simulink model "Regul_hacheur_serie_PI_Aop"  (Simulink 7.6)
settings: Solver=ode23tb  StartTime=0.0  StopTime=100  RelTol=1e-3
InitFcn:
  | clc, close all, clear all
  | rc=30;
  | 
  | Kp=1e-5; %1e-5 marche
  | R1=10e3;
  | R2=Kp*R1;
  | Ti=1e-4;
  | C=Ti/R2;
StopFcn:
  | clc
  | close all, clc
  | 
  | load csg_Imoy_charge.mat
  | figure
  | plot(x(1,:),x(2,:),x(1,:),x(3,:),x(1,:),x(4,:))
  | xlabel('temps')
  | title('Courant charge et Consigne')
  | grid
  | 
  | load err-cde-PID.mat
  | figure
  | plotyy(y(1,:),y(2,:),y(1,:),y(3,:))
  | xlabel('temps')
  | title('Erreur et Commande')
  | grid
  | 
  | delete *.mat
libraries: fl_lib x27, nesl_utility x13, powerlib x10, elec_lib x10, powerlib_extras x1

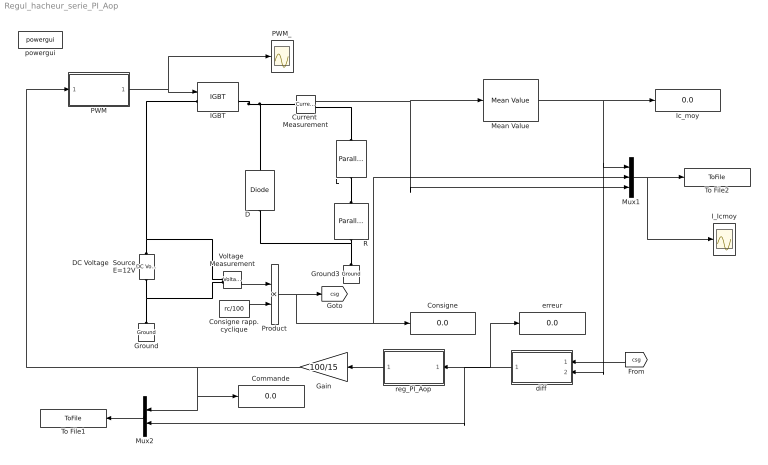
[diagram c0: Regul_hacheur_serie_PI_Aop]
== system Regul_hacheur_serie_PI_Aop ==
  Commande : Display
  Consigne : Display
  Consigne rapp. cyclique : Constant  Value=rc/100
  Current  Measurement : powerlib/Measurements/Current Measurement  DialogController=POWERSYS.PowerSysDialog  SystemSampleTime=-1  PhasorSimulation=off  OutputType=Complex  PSBequivalent=0
  D : powerlib/Power Electronics/Diode  DialogController=POWERSYS.PowerSysDialog  SystemSampleTime=-1  Ron=0.001  Lon=0  Vf=0.7  IC=0  UseSnubber=off  Rs=1e12  Cs=250e-12  Measurements=off
  DC Voltage  Source E=12V : powerlib/Electrical Sources/DC Voltage Source  DialogController=POWERSYS.PowerSysDialog  SystemSampleTime=-1  Amplitude=12  Measurements=None
  Gain : Gain  Gain=100/15
  Ground : powerlib/Elements/Ground  DialogController=POWERSYS.PowerSysDialog  PhysicalDomain=powersysdomain  SubClassName=unknown  LeftPortType=p1  RightPortType=p1  LConnTagsString=a
  Ground3 : powerlib/Elements/Ground  DialogController=POWERSYS.PowerSysDialog  PhysicalDomain=powersysdomain  SubClassName=unknown  LeftPortType=p1  RightPortType=p1  LConnTagsString=a
  IGBT : powerlib/Power Electronics/IGBT  DialogController=POWERSYS.PowerSysDialog  SystemSampleTime=-1  Ron=0.001  Lon=0  Vf=1  Tf=1e-6  Tt=2e-6  IC=0  Rs=1e5  Cs=inf  Measurements=on
  I_Icmoy : Scope
  Ic_moy : Display
  L : powerlib/Elements/Parallel RLC Branch  DialogController=POWERSYS.PowerSysDialog  PhysicalDomain=powersysdomain  SubClassName=unknown  LeftPortType=p1  RightPortType=p1  LConnTagsString=a  RConnTagsString=__new0  BranchType=L  Resistance=50  Inductance=10  SetiL0=off  InitialCurrent=0  Capacitance=25e-06  Setx0=off  InitialVoltage=0  Measurements=Branch voltage and current
  Mean Value : powerlib_extras/Measurements/Mean Value  DialogController=POWERSYS.PowerSysDialog  SystemSampleTime=-1  Period=10
  Mux1 : Mux  Inputs=3
  Mux2 : Mux  Inputs=2
  PWM : Subsystem
  PWM_ : Scope
  Product : Product
  R : powerlib/Elements/Parallel RLC Branch  DialogController=POWERSYS.PowerSysDialog  PhysicalDomain=powersysdomain  SubClassName=unknown  LeftPortType=p1  RightPortType=p1  LConnTagsString=a  RConnTagsString=__new0  BranchType=R  Resistance=1  Inductance=1.0  SetiL0=off  InitialCurrent=0  Capacitance=25e-06  Setx0=off  InitialVoltage=0  Measurements=Branch voltage and current
  To File1 : ToFile  Filename=err-cde-PID  MatrixName=y
  To File2 : ToFile  Filename=csg_Imoy_charge  MatrixName=x
  Voltage  Measurement : powerlib/Measurements/Voltage Measurement  DialogController=POWERSYS.PowerSysDialog  SystemSampleTime=-1  PhasorSimulation=off  OutputType=Complex  PSBequivalent=0
  diff : Subsystem
  erreur : Display
  powergui : powerlib/powergui  SystemSampleTime=-1  SimulationMode=Continuous  SampleTime=0  frequency=60  SPID=off  DisableSnubberDevices=off  DisableRonSwitches=off  DisableVfSwitches=off  SwTol=0  Interpol=off  frequencyindice=0  echomessages=off  HookPort=off  DisplayEquations=off  FunctionMessages=off  EnableUseOfTLC=off  x0status=blocks  RestoreLinks=warning  ResistiveCurrentMeasurement=off  Frange=[0:2:500]  Ylog=off  Xlog=on  ShowGrid=off  save=off  variable=ZData  ZoomFFT=on  StartTime=0.0  cycles=1  DisplayStyle=1  fundamental=60  FreqAxis=off  MaxFrequency=1000  frequencyindicesteady=1  RmsSteady=1  display=off  Ts=0  methode=off
  reg_PI_Aop : Subsystem
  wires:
  PWM/1(PWM) -> PWM_/1, IGBT/1
  Current  Measurement/1 -> Mean Value/1, Mux1/3
  Mean Value/1 -> Ic_moy/1, Mux1/1, diff/2(-I)
  Mux1/1 -> To File2/1, I_Icmoy/1
  Voltage  Measurement/1 -> Product/1
  Product/1 -> [csg], Consigne/1, Mux1/2
  Consigne rapp. cyclique/1 -> Product/2
  diff/1(err) -> erreur/1, Mux2/2, reg_PI_Aop/1(err)
  reg_PI_Aop/1(cde) -> Gain/1
  Mux2/1 -> To File1/1
  [csg] -> diff/1(+Csg)
  Gain/1 -> PWM/1(rc (%)), Commande/1, Mux2/1
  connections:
  DC Voltage  Source E=12V/LConn1 -- Ground/LConn1 -- Voltage  Measurement/LConn2
  DC Voltage  Source E=12V/RConn1 -- IGBT/LConn1 -- Voltage  Measurement/LConn1
  R/RConn1 -- Ground3/LConn1 -- D/LConn1
  IGBT/RConn1 -- D/RConn1 -- Current  Measurement/LConn1
  L/RConn1 -- R/LConn1
  L/LConn1 -- Current  Measurement/RConn1

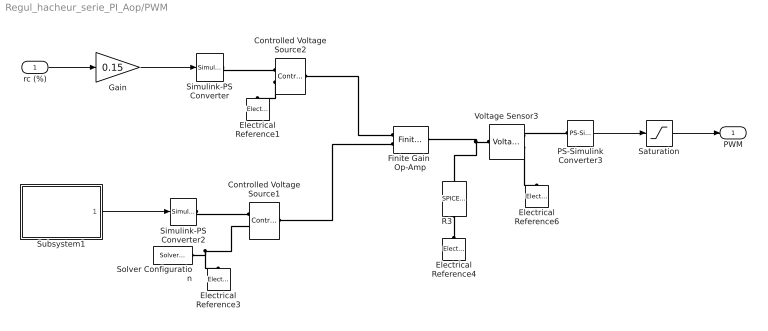
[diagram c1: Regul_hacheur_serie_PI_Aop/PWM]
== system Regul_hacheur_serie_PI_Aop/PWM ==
  rc (%) : Inport
  Controlled Voltage Source1 : fl_lib/Electrical/Electrical Sources/Controlled Voltage Source  DialogController=NetworkEngine.DynNeDlgSource  SystemSampleTime=-1  i_Log=off  v_Log=off  LocalVarNames=|current|voltage|power  LocalVarDescs=|Current (A)|Voltage (V)|Power (W)  LocalVarLogging=[0 0 0]
  Controlled Voltage Source2 : fl_lib/Electrical/Electrical Sources/Controlled Voltage Source  DialogController=NetworkEngine.DynNeDlgSource  SystemSampleTime=-1  i_Log=off  v_Log=off  LocalVarNames=|current|voltage|power  LocalVarDescs=|Current (A)|Voltage (V)|Power (W)  LocalVarLogging=[0 0 0]
  Electrical Reference{1,3..4,6} (4 alike) : fl_lib/Electrical/Electrical Elements/Electrical Reference  DialogController=NetworkEngine.DynNeDlgSource  SystemSampleTime=-1  i_Log=off  LocalVarNames=|i  LocalVarDescs=|i  LocalVarLogging=[]
  Finite Gain  Op-Amp : elec_lib/Integrated Circuits/Finite Gain Op-Amp  DialogController=NetworkEngine.DynNeDlgSource  SystemSampleTime=-1  A=1000  Rin=1e+06 Ohm  Rout=100 Ohm  Vmin=-12 V  Vmax=12 V  LocalVarNames=|power  LocalVarDescs=|Dissipated power (W)  LocalVarLogging=0
  Gain : Gain  Gain=0.15
  PS-Simulink Converter3 : nesl_utility/PS-Simulink Converter  DialogController=NetworkEngine.DynNeUtilDlgSource  SystemSampleTime=-1  PhysicalDomain=network_engine_domain  LeftPortType=input  RightPortType=output  SubClassName=ps_output  Unit=1  AffineConversion=off
  R3 : elec_lib/Additional Components/SPICE-Compatible Components/Passive Devices/SPICE Resistor  DialogController=NetworkEngine.DynNeDlgSource  SystemSampleTime=-1  SCALE=1  R_param=1  R=10e3 Ohm  RSH=0 Ohm  LENGTH=1e-06 m  WIDTH=1e-06 m  NARROW=0 m  T_param=1  TC1=0 1/K  TC2=0 1/K^2  TOFFSET=0 K  TFIXED=300.15 K  TMEAS=300.15 K  LocalVarLogging=[]
  Saturation : Saturate  UpperLimit=1  LowerLimit=0
  Simulink-PS Converter : nesl_utility/Simulink-PS Converter  DialogController=NetworkEngine.DynNeUtilDlgSource  SystemSampleTime=-1  PhysicalDomain=network_engine_domain  LeftPortType=input  RightPortType=output  SubClassName=ps_input  Unit=1  AffineConversion=off  InputFilterTimeConstant=.001  UdotUserProvided=0
  Simulink-PS Converter2 : nesl_utility/Simulink-PS Converter  DialogController=NetworkEngine.DynNeUtilDlgSource  SystemSampleTime=-1  PhysicalDomain=network_engine_domain  LeftPortType=input  RightPortType=output  SubClassName=ps_input  Unit=1  AffineConversion=off  InputFilterTimeConstant=.001  UdotUserProvided=0
  Solver Configuration : nesl_utility/Solver Configuration  DialogController=NetworkEngine.DynNeUtilDlgSource  SystemSampleTime=-1  PhysicalDomain=network_engine_domain  LeftPortType=input  RightPortType=generic  SubClassName=solver  Accelerate=off  Profile=off  ResidualTolerance=1e-12  MaxNonlinIter=12  MaxModeIter=2  DoFixedCost=on  UseLocalSampling=off  DoDC=off  LinearAlgebra=Sparse  LocalSolverSampleTime=.001  LocalSolverChoice=NE_BACKWARD_EULER_ADVANCER  UseLocalSolver=off
  Subsystem1 : Subsystem
  Voltage Sensor3 : fl_lib/Electrical/Electrical Sensors/Voltage Sensor  DialogController=NetworkEngine.DynNeDlgSource  SystemSampleTime=-1  i1_Log=off  v1_Log=off  LocalVarNames=|i1|v1  LocalVarDescs=|i1|v1  LocalVarLogging=[]
  PWM : Outport
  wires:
  Gain/1 -> Simulink-PS Converter/1
  Saturation/1 -> PWM/1
  PS-Simulink Converter3/1 -> Saturation/1
  rc (%)/1 -> Gain/1
  Subsystem1/1(tri) -> Simulink-PS Converter2/1
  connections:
  Voltage Sensor3/RConn1 -- PS-Simulink Converter3/LConn1
  Voltage Sensor3/LConn1 -- R3/RConn1 -- Finite Gain  Op-Amp/RConn1
  Voltage Sensor3/RConn2 -- Electrical Reference6/LConn1
  Electrical Reference4/LConn1 -- R3/LConn1
  Controlled Voltage Source2/RConn2 -- Electrical Reference1/LConn1
  Simulink-PS Converter/RConn1 -- Controlled Voltage Source2/RConn1
  Finite Gain  Op-Amp/LConn1 -- Controlled Voltage Source2/LConn1
  Solver Configuration/RConn1 -- Electrical Reference3/LConn1 -- Controlled Voltage Source1/RConn2
  Simulink-PS Converter2/RConn1 -- Controlled Voltage Source1/RConn1
  Controlled Voltage Source1/LConn1 -- Finite Gain  Op-Amp/LConn2

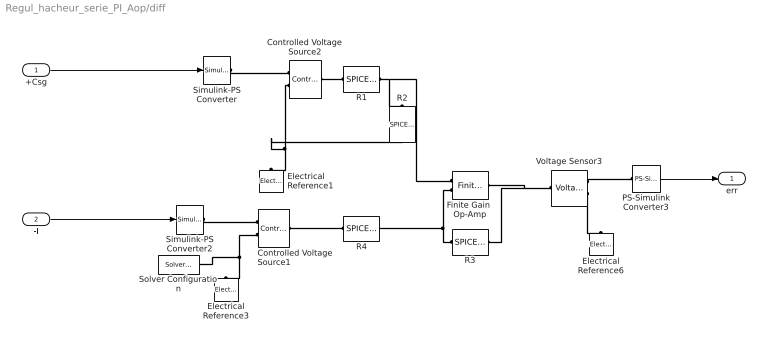
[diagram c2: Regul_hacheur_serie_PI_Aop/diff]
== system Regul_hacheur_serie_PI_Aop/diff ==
  +Csg : Inport
  -I : Inport  Port=2
  Controlled Voltage Source1 : fl_lib/Electrical/Electrical Sources/Controlled Voltage Source  DialogController=NetworkEngine.DynNeDlgSource  SystemSampleTime=-1  i_Log=off  v_Log=off  LocalVarNames=|current|voltage|power  LocalVarDescs=|Current (A)|Voltage (V)|Power (W)  LocalVarLogging=[0 0 0]
  Controlled Voltage Source2 : fl_lib/Electrical/Electrical Sources/Controlled Voltage Source  DialogController=NetworkEngine.DynNeDlgSource  SystemSampleTime=-1  i_Log=off  v_Log=off  LocalVarNames=|current|voltage|power  LocalVarDescs=|Current (A)|Voltage (V)|Power (W)  LocalVarLogging=[0 0 0]
  Electrical Reference1 : fl_lib/Electrical/Electrical Elements/Electrical Reference  DialogController=NetworkEngine.DynNeDlgSource  SystemSampleTime=-1  i_Log=off  LocalVarNames=|i  LocalVarDescs=|i  LocalVarLogging=[]
  Electrical Reference3 : fl_lib/Electrical/Electrical Elements/Electrical Reference  DialogController=NetworkEngine.DynNeDlgSource  SystemSampleTime=-1  i_Log=off  LocalVarNames=|i  LocalVarDescs=|i  LocalVarLogging=[]
  Electrical Reference6 : fl_lib/Electrical/Electrical Elements/Electrical Reference  DialogController=NetworkEngine.DynNeDlgSource  SystemSampleTime=-1  i_Log=off  LocalVarNames=|i  LocalVarDescs=|i  LocalVarLogging=[]
  Finite Gain  Op-Amp : elec_lib/Integrated Circuits/Finite Gain Op-Amp  DialogController=NetworkEngine.DynNeDlgSource  SystemSampleTime=-1  A=1000  Rin=1e+06 Ohm  Rout=100 Ohm  Vmin=-12 V  Vmax=12 V  LocalVarNames=|power  LocalVarDescs=|Dissipated power (W)  LocalVarLogging=0
  PS-Simulink Converter3 : nesl_utility/PS-Simulink Converter  DialogController=NetworkEngine.DynNeUtilDlgSource  SystemSampleTime=-1  PhysicalDomain=network_engine_domain  LeftPortType=input  RightPortType=output  SubClassName=ps_output  Unit=1  AffineConversion=off
  R{1..4} (4 alike) : elec_lib/Additional Components/SPICE-Compatible Components/Passive Devices/SPICE Resistor  DialogController=NetworkEngine.DynNeDlgSource  SystemSampleTime=-1  SCALE=1  R_param=1  R=10e3 Ohm  RSH=0 Ohm  LENGTH=1e-06 m  WIDTH=1e-06 m  NARROW=0 m  T_param=1  TC1=0 1/K  TC2=0 1/K^2  TOFFSET=0 K  TFIXED=300.15 K  TMEAS=300.15 K  LocalVarLogging=[]
  Simulink-PS Converter : nesl_utility/Simulink-PS Converter  DialogController=NetworkEngine.DynNeUtilDlgSource  SystemSampleTime=-1  PhysicalDomain=network_engine_domain  LeftPortType=input  RightPortType=output  SubClassName=ps_input  Unit=1  AffineConversion=off  InputFilterTimeConstant=.001  UdotUserProvided=0
  Simulink-PS Converter2 : nesl_utility/Simulink-PS Converter  DialogController=NetworkEngine.DynNeUtilDlgSource  SystemSampleTime=-1  PhysicalDomain=network_engine_domain  LeftPortType=input  RightPortType=output  SubClassName=ps_input  Unit=1  AffineConversion=off  InputFilterTimeConstant=.001  UdotUserProvided=0
  Solver Configuration : nesl_utility/Solver Configuration  DialogController=NetworkEngine.DynNeUtilDlgSource  SystemSampleTime=-1  PhysicalDomain=network_engine_domain  LeftPortType=input  RightPortType=generic  SubClassName=solver  Accelerate=off  Profile=off  ResidualTolerance=1e-12  MaxNonlinIter=12  MaxModeIter=2  DoFixedCost=on  UseLocalSampling=off  DoDC=off  LinearAlgebra=Sparse  LocalSolverSampleTime=.001  LocalSolverChoice=NE_BACKWARD_EULER_ADVANCER  UseLocalSolver=off
  Voltage Sensor3 : fl_lib/Electrical/Electrical Sensors/Voltage Sensor  DialogController=NetworkEngine.DynNeDlgSource  SystemSampleTime=-1  i1_Log=off  v1_Log=off  LocalVarNames=|i1|v1  LocalVarDescs=|i1|v1  LocalVarLogging=[]
  err : Outport
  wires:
  -I/1 -> Simulink-PS Converter2/1
  +Csg/1 -> Simulink-PS Converter/1
  PS-Simulink Converter3/1 -> err/1
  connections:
  Simulink-PS Converter2/RConn1 -- Controlled Voltage Source1/RConn1
  Controlled Voltage Source1/RConn2 -- Electrical Reference3/LConn1 -- Solver Configuration/RConn1
  Simulink-PS Converter/RConn1 -- Controlled Voltage Source2/RConn1
  Controlled Voltage Source2/RConn2 -- Electrical Reference1/LConn1 -- R2/RConn1
  Voltage Sensor3/RConn2 -- Electrical Reference6/LConn1
  R3/RConn1 -- Finite Gain  Op-Amp/RConn1 -- Voltage Sensor3/LConn1
  Voltage Sensor3/RConn1 -- PS-Simulink Converter3/LConn1
  R1/LConn1 -- Controlled Voltage Source2/LConn1
  R1/RConn1 -- R2/LConn1 -- Finite Gain  Op-Amp/LConn1
  R3/LConn1 -- Finite Gain  Op-Amp/LConn2 -- R4/RConn1
  Controlled Voltage Source1/LConn1 -- R4/LConn1

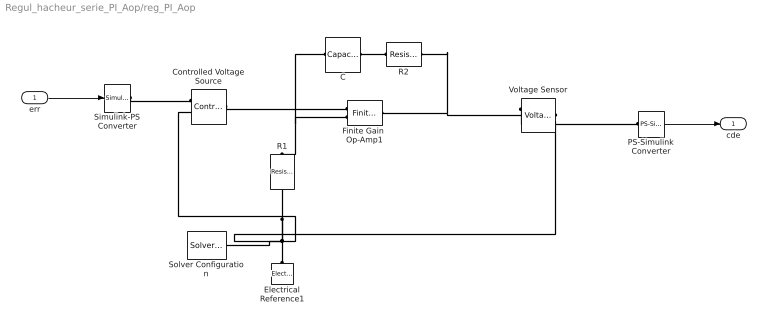
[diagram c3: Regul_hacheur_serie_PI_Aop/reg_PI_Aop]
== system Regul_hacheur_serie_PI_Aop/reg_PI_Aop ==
  err : Inport
  C : fl_lib/Electrical/Electrical Elements/Capacitor  DialogController=NetworkEngine.DynNeDlgSource  SystemSampleTime=-1  c=C F  v0=0 V  r=1e-6 Ohm  g=0 1/Ohm  i_Log=off  v_Log=off  vc_Log=off  LocalVarNames=|i|v|vc  LocalVarDescs=|i|v|Internal variable for voltage across capacitor term  LocalVarLogging=[0 0 0]
  Controlled Voltage Source : fl_lib/Electrical/Electrical Sources/Controlled Voltage Source  DialogController=NetworkEngine.DynNeDlgSource  SystemSampleTime=-1  i_Log=off  v_Log=off  LocalVarNames=|i|v  LocalVarDescs=|i|v  LocalVarLogging=[0 0]
  Electrical Reference1 : fl_lib/Electrical/Electrical Elements/Electrical Reference  DialogController=NetworkEngine.DynNeDlgSource  SystemSampleTime=-1  i_Log=off  LocalVarNames=|i  LocalVarDescs=|i  LocalVarLogging=[]
  Finite Gain  Op-Amp1 : elec_lib/Integrated Circuits/Finite Gain Op-Amp  DialogController=NetworkEngine.DynNeDlgSource  SystemSampleTime=-1  A=1000  Rin=1e+6 Ohm  Rout=100 Ohm  Vmin=-15 V  Vmax=15 V  LocalVarLogging=[]
  PS-Simulink Converter : nesl_utility/PS-Simulink Converter  DialogController=NetworkEngine.DynNeUtilDlgSource  SystemSampleTime=-1  PhysicalDomain=network_engine_domain  LeftPortType=input  RightPortType=output  SubClassName=ps_output  Unit=1  AffineConversion=off
  R1 : fl_lib/Electrical/Electrical Elements/Resistor  DialogController=NetworkEngine.DynNeDlgSource  SystemSampleTime=-1  R=R1 Ohm  i_Log=off  v_Log=off  LocalVarNames=|current|voltage|power  LocalVarDescs=|Resistor current (A)|Voltage across resistor (V)|Power (W)  LocalVarLogging=[0 0 0]
  R2 : fl_lib/Electrical/Electrical Elements/Resistor  DialogController=NetworkEngine.DynNeDlgSource  SystemSampleTime=-1  R=R2 Ohm  i_Log=off  v_Log=off  LocalVarNames=|current|voltage|power  LocalVarDescs=|Resistor current (A)|Voltage across resistor (V)|Power (W)  LocalVarLogging=[0 0 0]
  Simulink-PS Converter : nesl_utility/Simulink-PS Converter  DialogController=NetworkEngine.DynNeUtilDlgSource  SystemSampleTime=-1  PhysicalDomain=network_engine_domain  LeftPortType=input  RightPortType=output  SubClassName=ps_input  Unit=1  AffineConversion=off  InputFilterTimeConstant=.001  UdotUserProvided=0
  Solver Configuration : nesl_utility/Solver Configuration  DialogController=NetworkEngine.DynNeUtilDlgSource  SystemSampleTime=-1  PhysicalDomain=network_engine_domain  LeftPortType=input  RightPortType=generic  SubClassName=solver  Accelerate=off  Profile=off  ResidualTolerance=1e-9  MaxNonlinIter=3  MaxModeIter=2  DoFixedCost=off  UseLocalSampling=off  DoDC=off  LinearAlgebra=Sparse  LocalSolverSampleTime=.001  LocalSolverChoice=NE_BACKWARD_EULER_ADVANCER  UseLocalSolver=off
  Voltage Sensor : fl_lib/Electrical/Electrical Sensors/Voltage Sensor  DialogController=NetworkEngine.DynNeDlgSource  SystemSampleTime=-1  i1_Log=off  v1_Log=off  LocalVarNames=|i1|v1  LocalVarDescs=|i1|v1  LocalVarLogging=[0 0]
  cde : Outport
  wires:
  PS-Simulink Converter/1 -> cde/1
  err/1 -> Simulink-PS Converter/1
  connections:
  C/LConn1 -- R1/RConn1 -- Finite Gain  Op-Amp1/LConn2
  C/RConn1 -- R2/LConn1
  R1/LConn1 -- Voltage Sensor/RConn2 -- Controlled Voltage Source/RConn2 -- Electrical Reference1/LConn1 -- Solver Configuration/RConn1
  Finite Gain  Op-Amp1/RConn1 -- R2/RConn1 -- Voltage Sensor/LConn1
  Voltage Sensor/RConn1 -- PS-Simulink Converter/LConn1
  Simulink-PS Converter/RConn1 -- Controlled Voltage Source/RConn1
  Controlled Voltage Source/LConn1 -- Finite Gain  Op-Amp1/LConn1

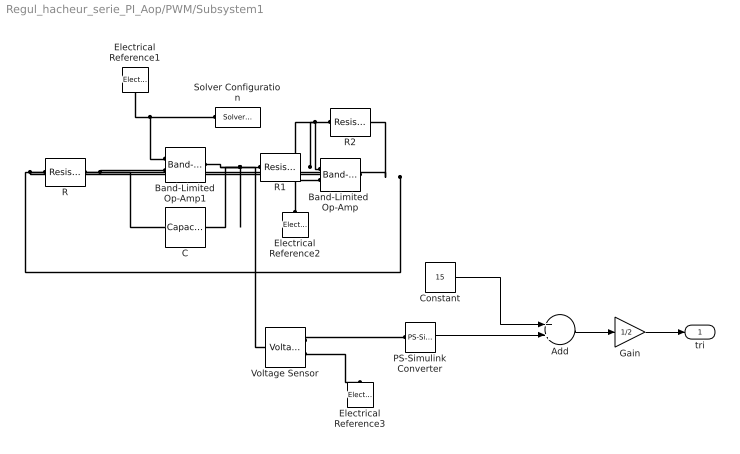
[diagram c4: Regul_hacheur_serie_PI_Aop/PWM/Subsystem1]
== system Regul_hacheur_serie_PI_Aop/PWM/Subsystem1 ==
  Add : Sum
  Band-Limited  Op-Amp : elec_lib/Integrated Circuits/Band-Limited Op-Amp  DialogController=NetworkEngine.DynNeDlgSource  SystemSampleTime=-1  A=1000  Rin=1e+06 Ohm  Rout=100 Ohm  Vmin=-15 V  Vmax=15 V  Vdotmax=1000 V/s  f=1e+05 Hz  V0=0 V  LocalVarNames=|power  LocalVarDescs=|Dissipated power (W)  LocalVarLogging=0
  Band-Limited Op-Amp1 : elec_lib/Integrated Circuits/Band-Limited Op-Amp  DialogController=NetworkEngine.DynNeDlgSource  SystemSampleTime=-1  A=1000  Rin=1e+06 Ohm  Rout=100 Ohm  Vmin=-15 V  Vmax=15 V  Vdotmax=1000 V/s  f=1e+05 Hz  V0=0 V  LocalVarNames=|power  LocalVarDescs=|Dissipated power (W)  LocalVarLogging=0
  C : fl_lib/Electrical/Electrical Elements/Capacitor  DialogController=NetworkEngine.DynNeDlgSource  SystemSampleTime=-1  c=0.1e-5 F  v0=0.1 V  r=1e-6 Ohm  g=0 1/Ohm  i_Log=off  v_Log=off  vc_Log=off  LocalVarNames=|current|voltage|power  LocalVarDescs=|Capacitor current (A)|Voltage across capacitor (V)|Power (W)  LocalVarLogging=[0 0 0]
  Constant : Constant  Value=15
  Electrical Reference1 : fl_lib/Electrical/Electrical Elements/Electrical Reference  DialogController=NetworkEngine.DynNeDlgSource  SystemSampleTime=-1  i_Log=off  LocalVarNames=|i  LocalVarDescs=|i  LocalVarLogging=[]
  Electrical Reference2 : fl_lib/Electrical/Electrical Elements/Electrical Reference  DialogController=NetworkEngine.DynNeDlgSource  SystemSampleTime=-1  i_Log=off  LocalVarNames=|i  LocalVarDescs=|i  LocalVarLogging=[]
  Electrical Reference3 : fl_lib/Electrical/Electrical Elements/Electrical Reference  DialogController=NetworkEngine.DynNeDlgSource  SystemSampleTime=-1  i_Log=off  LocalVarNames=|i  LocalVarDescs=|i  LocalVarLogging=[]
  Gain : Gain  Gain=1/2
  PS-Simulink Converter : nesl_utility/PS-Simulink Converter  DialogController=NetworkEngine.DynNeUtilDlgSource  SystemSampleTime=-1  PhysicalDomain=network_engine_domain  LeftPortType=input  RightPortType=output  SubClassName=ps_output  Unit=1  AffineConversion=off
  R : fl_lib/Electrical/Electrical Elements/Resistor  DialogController=NetworkEngine.DynNeDlgSource  SystemSampleTime=-1  R=1000 Ohm  i_Log=off  v_Log=off  LocalVarNames=|current|voltage|power  LocalVarDescs=|Resistor current (A)|Voltage across resistor (V)|Power (W)  LocalVarLogging=[0 0 0]
  R1 : fl_lib/Electrical/Electrical Elements/Resistor  DialogController=NetworkEngine.DynNeDlgSource  SystemSampleTime=-1  R=10e3 Ohm  i_Log=off  v_Log=off  LocalVarNames=|current|voltage|power  LocalVarDescs=|Resistor current (A)|Voltage across resistor (V)|Power (W)  LocalVarLogging=[0 0 0]
  R2 : fl_lib/Electrical/Electrical Elements/Resistor  DialogController=NetworkEngine.DynNeDlgSource  SystemSampleTime=-1  R=10e3 Ohm  i_Log=off  v_Log=off  LocalVarNames=|current|voltage|power  LocalVarDescs=|Resistor current (A)|Voltage across resistor (V)|Power (W)  LocalVarLogging=[0 0 0]
  Solver Configuration : nesl_utility/Solver Configuration  DialogController=NetworkEngine.DynNeUtilDlgSource  SystemSampleTime=-1  PhysicalDomain=network_engine_domain  LeftPortType=input  RightPortType=generic  SubClassName=solver  Accelerate=off  Profile=off  ResidualTolerance=1e-9  MaxNonlinIter=12  MaxModeIter=2  DoFixedCost=off  UseLocalSampling=off  DoDC=off  LinearAlgebra=Sparse  LocalSolverSampleTime=.001  LocalSolverChoice=NE_BACKWARD_EULER_ADVANCER  UseLocalSolver=off
  Voltage Sensor : fl_lib/Electrical/Electrical Sensors/Voltage Sensor  DialogController=NetworkEngine.DynNeDlgSource  SystemSampleTime=-1  i1_Log=off  v1_Log=off  LocalVarNames=|i1|v1  LocalVarDescs=|i1|v1  LocalVarLogging=[]
  tri : Outport
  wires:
  PS-Simulink Converter/1 -> Add/2
  Constant/1 -> Add/1
  Add/1 -> Gain/1
  Gain/1 -> tri/1
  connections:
  Voltage Sensor/RConn1 -- PS-Simulink Converter/LConn1
  Band-Limited Op-Amp1/RConn1 -- R1/LConn1 -- C/RConn1 -- Voltage Sensor/LConn1
  R/RConn1 -- C/LConn1 -- Band-Limited Op-Amp1/LConn2
  Solver Configuration/RConn1 -- Band-Limited Op-Amp1/LConn1 -- Electrical Reference1/LConn1
  R/LConn1 -- Band-Limited  Op-Amp/RConn1 -- R2/RConn1
  Electrical Reference2/LConn1 -- Band-Limited  Op-Amp/LConn2
  R2/LConn1 -- Band-Limited  Op-Amp/LConn1 -- R1/RConn1
  Voltage Sensor/RConn2 -- Electrical Reference3/LConn1
